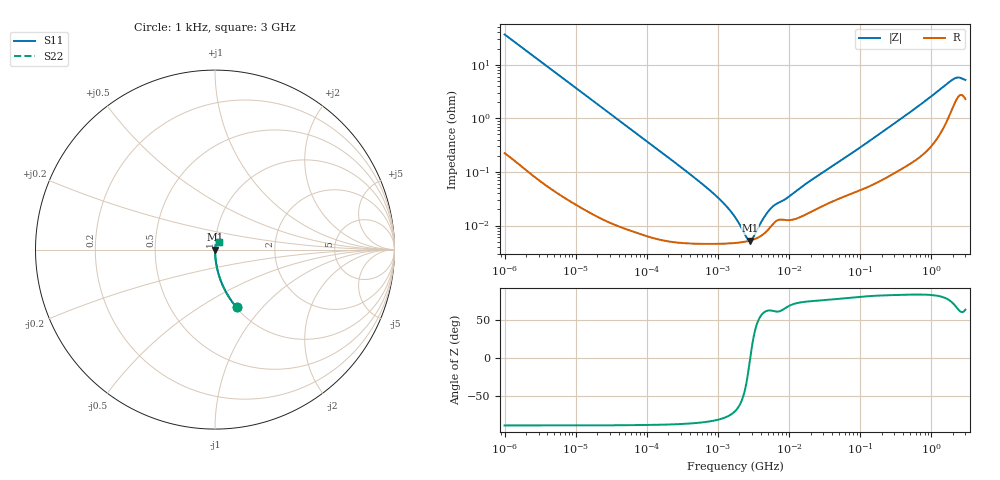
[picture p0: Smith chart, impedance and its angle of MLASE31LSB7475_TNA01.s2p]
! MLASE31LSB7475_TNA01  S-PARAMETER MODEL  ( Standard Model )
! Model Generated by TAIYO YUDEN Corporation (http://www.ty-top.com)
! Version 2.0
! TAIYO YUDEN Control No. 240510
! Copyright(c) 2014 TAIYO YUDEN CO.,LTD. All Rights Reserved.
! Product Description (link to TY-COMPAS)
! https://ds.yuden.co.jp/TYCOMPAS/or/detail?pn=MLASE31LSB7475KTNA01&u=M
! Products Name : Multilayer Ceramic Capacitors
! Characteristics :
!  Capacitance : 4.7 [uF] , Rated Voltage : 16 [V] , TCC : X7R
!  Case Size : 3.2 x 1.6 / 0.126 x 0.063 [mm/inch] , Thickness : 1.6 / 0.063 [mm/inch]
!  (Conditions: Temperature = 25 [degC] , DC Bias Voltage = 0 [V])
! External Node Assignments :
!  1  o---| |---o  2
! GND o---------o GND
! Frequency Range : 1kHz  -  3GHz  [ 401 STEP ]
# MHZ S RI R 50
! Freq[MHz].  S11 Real  S11 Imag  S21 Real  S21 Imag  S12 Real  S12 Imag  S22 Real  S22 Imag
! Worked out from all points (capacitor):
!   401 points, 1 kHz to 3 GHz, reference 50 ohm
!   read as one part in series: C = 4.33 uF near 1.077 kHz
!   lowest |Z| = 5.26 mohm at 2.812 MHz (marker M1)
!   series resonance near 2.84 MHz, so ESL is about 730 pH
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0.001  0.1201 -0.3221  0.8799 0.3221  0.8799 0.3221  0.1201 -0.3221
0.001685  0.0466 -0.2078  0.9534 0.2078  0.9534 0.2078  0.0466 -0.2078
0.00306  0.015 -0.1185  0.985 0.1185  0.985 0.1185  0.015 -0.1185
0.005768  0.00446 -0.0637  0.9955 0.0637  0.9955 0.0637  0.00446 -0.0637
0.01216  0.00114 -0.0304  0.9989 0.0304  0.9989 0.0304  0.00114 -0.0304
0.147855  6.12e-05 -0.00252  0.9999 0.00252  0.9999 0.00252  6.12e-05 -0.00252
0.43594  4.68e-05 -0.000839  1 0.000839  1 0.000839  4.68e-05 -0.000839
0.821683  4.57e-05 -0.000418  1 0.000418  1 0.000418  4.57e-05 -0.000418
1.285341  4.62e-05 -0.000232  1 0.000232  1 0.000232  4.62e-05 -0.000232
1.732051  4.74e-05 -0.000136  1 0.000136  1 0.000136  4.74e-05 -0.000136
2.087011  4.87e-05 -8.3e-05  1 8.3e-05  1 8.3e-05  4.87e-05 -8.3e-05
2.812335  5.25e-05 -2.56e-06  0.9999 2.56e-06  0.9999 2.56e-06  5.25e-05 -2.56e-06
3.517417  5.83e-05 5.78e-05  0.9999 -5.78e-05  0.9999 -5.78e-05  5.83e-05 5.78e-05
3.789741  6.13e-05 7.86e-05  0.9999 -7.86e-05  0.9999 -7.86e-05  6.13e-05 7.86e-05
4.919932  8.05e-05 0.000154  0.9999 -0.000154  0.9999 -0.000154  8.05e-05 0.000154
5.928204  0.000107 0.000203  0.9999 -0.000203  0.9999 -0.000203  0.000107 0.000203
9.273352  0.000126 0.0003  0.9999 -0.0003  0.9999 -0.0003  0.000126 0.0003
21.06097  0.000186 0.000701  0.9998 -0.000701  0.9998 -0.000701  0.000186 0.000701
256.0921  0.000886 0.00685  0.9991 -0.00685  0.9991 -0.00685  0.000886 0.00685
1990.675  0.018 0.0488  0.982 -0.0488  0.982 -0.0488  0.018 0.0488
2398.636  0.0274 0.0492  0.9726 -0.0492  0.9726 -0.0492  0.0274 0.0492
3000  0.0244 0.0444  0.9756 -0.0444  0.9756 -0.0444  0.0244 0.0444
